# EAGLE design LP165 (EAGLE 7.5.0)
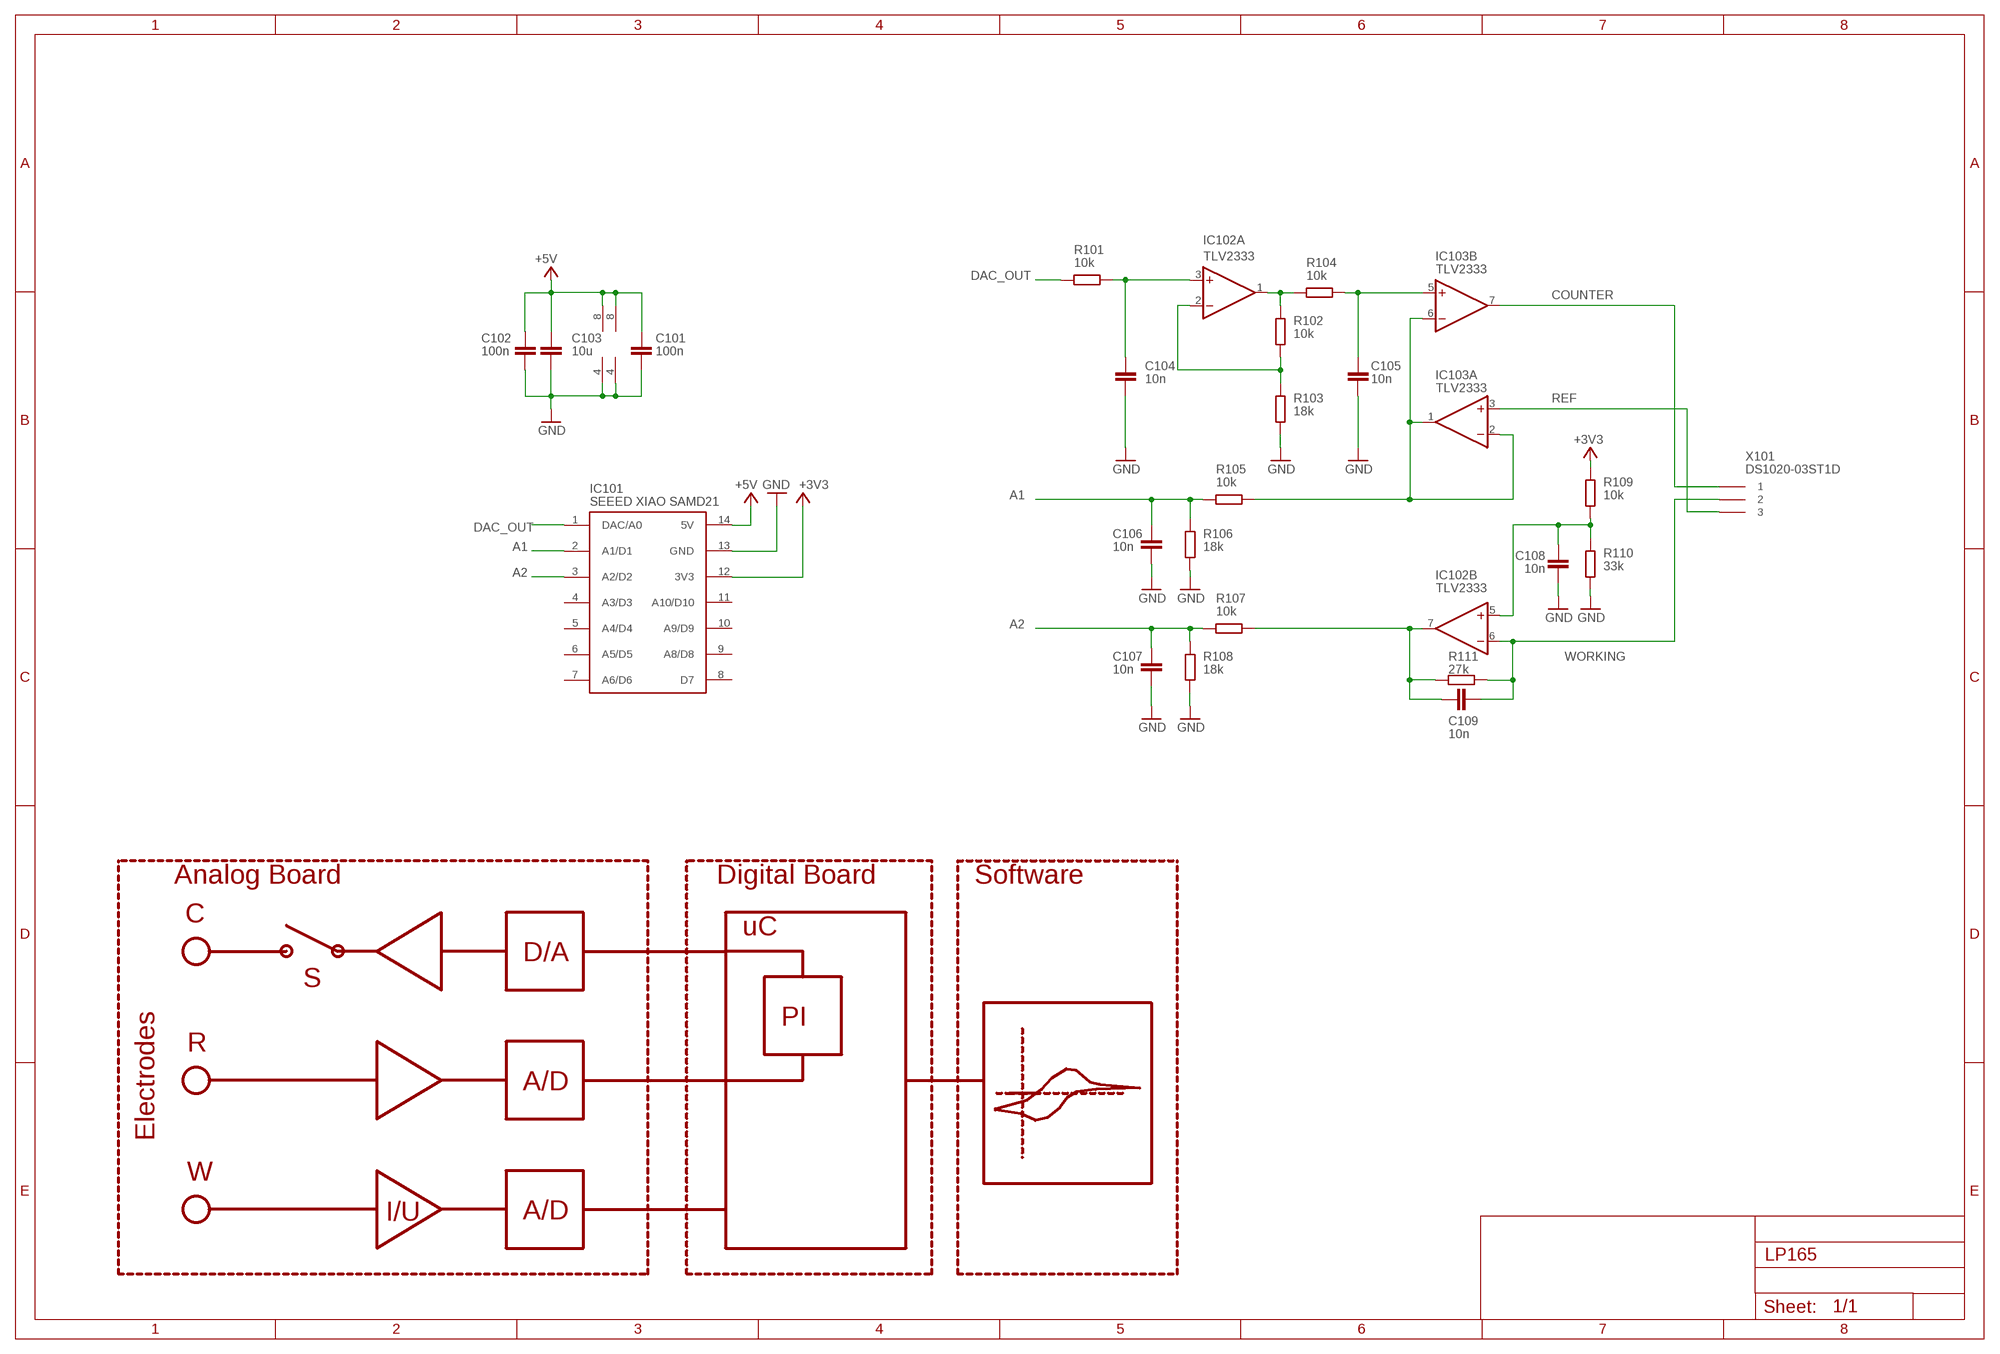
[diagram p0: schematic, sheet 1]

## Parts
C101  100n  C-EUC0805  [C0805]
C102  100n  C-EUC0805  [C0805]
C103  10u  C-EUC0805  [C0805]
C104  10n  C-EUC0805  [C0805]
C105  10n  C-EUC0805  [C0805]
C106  10n  C-EUC0805  [C0805]
C107  10n  C-EUC0805  [C0805]
C108  10n  C-EUC0805  [C0805]
C109  10n  C-EUC0805  [C0805]
IC101  SEEED XIAO SAMD21  SEEED_XIAO  [SEEEDXIAO]
IC102  TLV2333  TLV2333IDR  [SO8]
IC103  TLV2333  TLV2333IDR  [SO8]
R101  10k  R-EU_R0805  [R0805]
R102  10k  R-EU_R0805  [R0805]
R103  18k  R-EU_R0805  [R0805]
R104  10k  R-EU_R0805  [R0805]
R105  10k  R-EU_R0805  [R0805]
R106  18k  R-EU_R0805  [R0805]
R107  10k  R-EU_R0805  [R0805]
R108  18k  R-EU_R0805  [R0805]
R109  10k  R-EU_R0805  [R0805]
R110  33k  R-EU_R0805  [R0805]
R111  27k  R-EU_R0805  [R0805]
X101  DS1020-03ST1D  [DS1020-03ST1D]

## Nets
+3V3: IC101.12(3V3) R109.2
+5V: C101.1 C102.1 C103.1 IC101.14(5V) IC102.8(P:V+) IC103.8(P:V+)
A1: C106.1 IC101.2(A1/D1) R105.1 R106.2
A2: C107.1 IC101.3(A2/D2) R107.1 R108.2
COUNTER: IC103.7(B:OUT) X101.1
DAC_OUT: IC101.1(DAC/A0) R101.1
GND: C101.2 C102.2 C103.2 C104.2 C105.2 C106.2 C107.2 C108.1 IC101.13(GND) IC102.4(P:V-) IC103.4(P:V-) R103.1 R106.1 R108.1 R110.2
N$2: C104.1 IC102.3(A:+IN) R101.2
N$5: IC102.1(A:OUT) R102.2 R104.1
N$6: C105.1 IC103.5(B:+IN) R104.2
N$7: IC102.2(A:-IN) R102.1 R103.2
N$8: IC103.1(A:OUT) IC103.2(A:-IN) IC103.6(B:-IN) R105.2
N$11: C109.1 IC102.7(B:OUT) R107.2 R111.1
N$18: C108.2 IC102.5(B:+IN) R109.1 R110.1
REF: IC103.3(A:+IN) X101.3
WORKING: C109.2 IC102.6(B:-IN) R111.2 X101.2
Unconnected: IC101.4(A3/D3) IC101.5(A4/D4) IC101.6(A5/D5) IC101.7(A6/D6) IC101.8(D7) IC101.9(A8/D8) IC101.10(A9/D9) IC101.11(A10/D10)

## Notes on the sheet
- Analog Board | Digital Board | Software
- C
- uC
- D/A
- S
- PI
- R
- A/D
- Electrodes
- W
- I/U | A/D

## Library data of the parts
C101-C109 = rcl:C-EU: CAPACITOR, European symbol
IC101 = user _eagleV7:SEEED_XIAO
IC102 IC103 = user _eagleV7:TLV2333IDR
R101-R111 = rcl:R-EU_: RESISTOR, European symbol
X101 = user _eagleV7:DS1020-03ST1D: Conrad: 1389988 Hst.-Teile-Nr.: DS1020-03ST1D

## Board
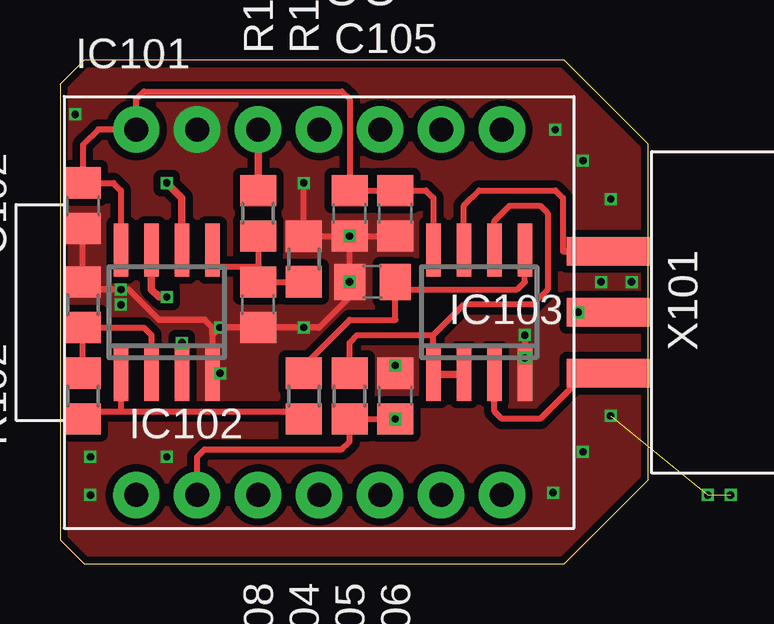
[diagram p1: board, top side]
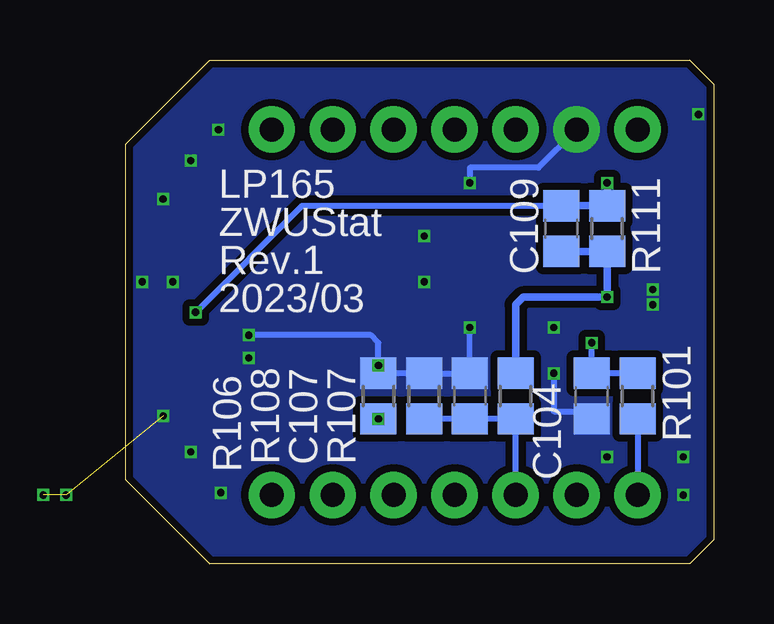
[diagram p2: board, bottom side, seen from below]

Size 24.5 x 21 mm. Coordinates in mm from the lower left corner, seen from the top.
Outline: 1,0 21,0 24.5,3.5 24.5,17.5 21,21 1,21 0,20 0,1 1,0
Copper layers (1*16): Top 0.018mm / dielectric 1.55mm / Bottom 0.018mm
Design rules "Multi-CB_2L_100µm-Tracks_OL35µm": minimum track width 0.1mm, minimum drill 0.2mm, track to track 0.1mm, track to pad 0.1mm, pad to pad 0.1mm, via to via 0.1mm, smd to smd 0mil, copper to edge 0.2mm, drill to drill 0.2mm, minimum pad ring 0.125mm, minimum via ring 0.1mm, stop-mask expansion 2mil, vias tented up to drill 0.45mm, thermal gap 0.2mm

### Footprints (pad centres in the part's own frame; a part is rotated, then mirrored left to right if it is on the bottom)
C0805 = smd 1.3 x 1.5: 1 -0.95,0; 2 0.95,0
SEEEDXIAO = drill 1 pad 1.93: 1 -7.62,-7.62; 2 -5.08,-7.62; 3 -2.54,-7.62; 4 0,-7.62; 5 2.54,-7.62; 6 5.08,-7.62; 7 7.62,-7.62; 8 7.62,7.62; 9 5.08,7.62; 10 2.54,7.62; 11 0,7.62; 12 -2.54,7.62; 13 -5.08,7.62; 14 -7.62,7.62
SO8 = smd 0.6 x 2.2: 1 -1.905,-2.6; 2 -0.635,-2.6; 3 0.635,-2.6; 4 1.905,-2.6; 5 1.905,2.6; 6 0.635,2.6; 7 -0.635,2.6; 8 -1.905,2.6
R0805 = smd 1.3 x 1.5: 1 -0.95,0; 2 0.95,0
DS1020-03ST1D = smd 3.5 x 1.2: 1 0,2.54; 2 0,0; 3 0,-2.54

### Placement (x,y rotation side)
C101  13.97,14.61 270 top
C102  0.95,14.92 270 top
C103  12.06,14.61 270 top
C104  5.08,6.99 270 bottom
C105  13.02,11.75 180 top
C106  13.97,6.99 90 top
C107  10.16,6.99 90 bottom
C108  8.26,10.79 90 top
C109  6.35,13.97 90 bottom
IC101  10.79,10.48 0 top
IC102  4.45,10.48 0 top
IC103  17.46,10.48 0 top
R101  3.17,6.99 90 bottom
R102  0.95,6.99 270 top
R103  0.95,10.79 270 top
R104  10.16,6.99 90 top
R105  12.06,6.99 90 top
R106  13.97,6.99 270 bottom
R107  8.26,6.99 90 bottom
R108  12.06,6.99 270 bottom
R109  8.26,14.61 90 top
R110  10.16,12.7 90 top
R111  4.45,13.97 90 bottom
X101  22.86,10.48 0 top

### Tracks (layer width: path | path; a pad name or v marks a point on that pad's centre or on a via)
+3V3
  Top 0.305: IC101.12 R109.2
+5V
  Top 0.254: IC102.8 2.54,15.56 2.23,15.87 C102.1 0.95,17.46 1.59,18.1 IC101.14 3.17,19.37 3.49,19.68 11.75,19.68 12.06,19.37 C103.1 C101.1 15.24,15.55 15.56,15.24 IC103.8
A1  (via drill 0.3)
  Top 0.254: IC101.2 5.71,4.45 6.03,4.76 11.75,4.76 12.06,5.08 R105.1 C106.1 v13.97,6.03
  Bottom 0.254: C106.1 v13.97,6.03
A2
  Bottom 0.254: IC101.3 R107.1 C107.1 R108.2
COUNTER
  Top 0.254: IC103.7 16.83,14.92 17.46,15.56 20.64,15.56 20.95,15.24 20.95,13.02 X101.1
DAC_OUT
  Bottom 0.254: R101.1 IC101.1
GND  (via drill 0.3)  (2 unrouted)
  Top 0.254: v12.06,13.65 C101.2 | v12.06,13.65 R110.2 v10.16,15.88 | 6.35,9.53 v6.67,9.85 C108.1 v10.16,9.84 10.79,9.84 12.07,11.12 C105.2 v12.07,13.65 v12.06,13.65 | 6.35,9.53 6.35,7.94 | v13.97,8.26 R106.1 | 6.35,9.53 6.35,9.84 6.03,10.16 4.13,10.16 2.86,11.43 1.27,11.43 R103.1 C102.2 | v19.37,9.53 IC103.4 | IC102.4 6.35,7.94 | 6.35,7.94 v6.67,7.94
  Bottom 0.254: R106.1 R108.1 C107.2 v10.16,9.84 | R106.1 v13.97,8.26 | R106.1 13.97,9.21 14.29,9.53 v19.37,9.53 | v6.67,7.94 6.67,6.35 5.4,6.35 5.08,5.71 C104.2 | IC101.13 7.3,16.51 10.16,16.51 v10.16,15.88
  other vias: 20.64,18.1 21.79,16.8 22.94,15.2 23.81,11.75 22.54,11.75 27.94,2.86 26.99,2.86 22.94,6.16 21.79,4.66 20.54,2.96 19.37,8.57 12.06,11.75 2.54,11.43 0.64,18.73 1.27,4.45 1.27,2.86 4.45,4.45 2.54,10.79
  pour Top (isolate 0.305, no thermals): -1.27,21.27 25.08,21.27 25.08,-0.32 -1.27,-0.32
  pour Bottom (isolate 0.305, no thermals): -1.27,21.27 25.08,21.27 25.08,-0.32 -1.27,-0.32
N$2  (via drill 0.3)
  Top 0.254: v5.08,9.21 IC102.3
  Bottom 0.254: R101.2 C104.1 v5.08,9.21
N$5
  Top 0.254: IC102.1 2.54,6.35 | 2.54,6.35 10.16,6.35 R104.1 | R102.2 1.27,6.35 2.54,6.35
N$6
  Top 0.254: R104.2 9.84,7.93 12.06,10.16 13.97,10.16 13.97,11.43 | 13.97,11.43 C105.1 13.97,11.43 | 13.97,11.43 19.05,11.43 19.37,11.75 IC103.5
N$7
  Top 0.254: R102.1 R103.2 | R103.2 3.49,9.84 3.81,9.53 IC102.2
  Top 0.406: R103.2
N$8
  Top 0.254: IC103.6 18.1,14.29 18.73,14.92 20,14.92 20.32,14.61 20.32,11.43 19.68,10.79 16.83,10.79 15.56,9.53 | R105.2 12.06,9.21 12.38,9.53 15.56,9.53 | IC103.1 15.56,9.53
  Top 0.305: IC103.1 IC103.2
N$11  (via drill 0.3)
  Top 0.305: v4.45,11.11 4.13,11.11 3.81,11.43 IC102.7
  Bottom 0.305: C109.1 R111.1 v4.45,11.11 7.94,11.11 8.26,10.79 R107.2
N$18
  Top 0.254: 6.35,12.38 8.25,12.38 | R109.1 8.26,12.38 | C108.2 R110.1
  Top 0.305: IC102.5 6.35,12.38 | C108.2 8.25,12.38 8.26,12.38
REF
  Top 0.254: X101.3 21.91,7.94 20,6.03 18.41,6.03 18.1,6.35 IC103.3
WORKING  (via drill 0.3)
  Top 0.254: v21.59,10.48 X101.2
  Top 0.305: v4.45,15.88 5.08,15.24 IC102.6
  Bottom 0.254: C109.2 17.14,14.92 v21.59,10.48
  Bottom 0.305: v4.45,15.88 R111.2 C109.2

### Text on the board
bNames: LP165 | ZWUStat | Rev.1 | 2023/03
Document: CE | WE | REF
